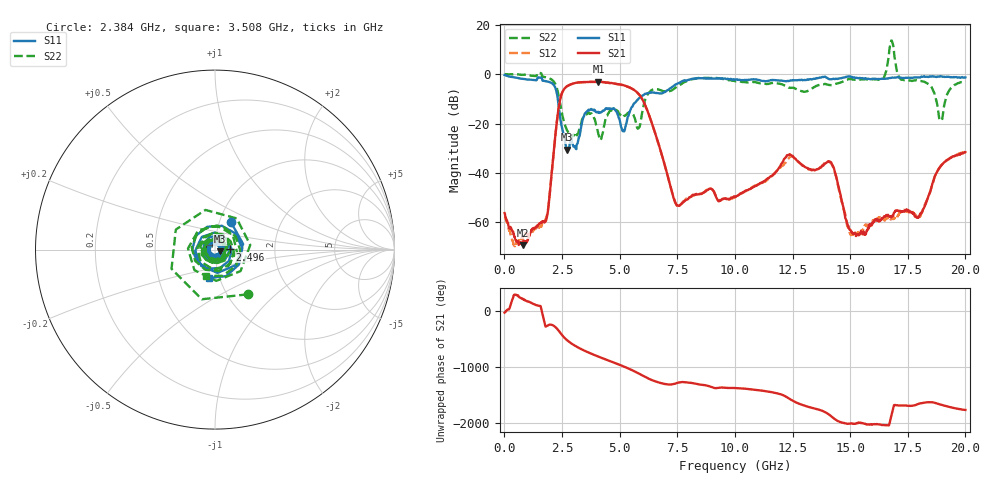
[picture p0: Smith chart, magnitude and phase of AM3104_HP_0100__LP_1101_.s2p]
!Created with skrf (http://scikit-rf.org).
# Hz S RI R 50.0
!freq ReS11 ImS11 ReS21 ImS21 ReS12 ImS12 ReS22 ImS22
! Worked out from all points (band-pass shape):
!   1601 points, 10 MHz to 20 GHz, reference 50 ohm
!   highest |S21| = -3.10 dB at 4.083 GHz (marker M1); lowest = -69.2 dB at 797.1 MHz (marker M2)
!   |S21| within 3 dB of the highest: 2.589 GHz to 5.576 GHz (2.987 GHz wide, 73.2 % of centre)
!   lowest |S11| = -30.6 dB at 2.721 GHz (marker M3), VSWR 1.06, Z = 52.9 - j0.943 ohm
!   |S11| at or under -10 dB: 2.316 GHz to 5.816 GHz (3.5 GHz wide, 86.1 % of centre)
!   |S22| runs from -26.8 to 13.6 dB; largest |S21 - S12| = 0.071
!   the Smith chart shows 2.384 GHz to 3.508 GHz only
!   S11 on the Smith chart (normalised r, x): 2.384 GHz: 1.13, +0.36; 2.496 GHz: 1.18, +0.00; 3.508 GHz: 0.89, -0.29
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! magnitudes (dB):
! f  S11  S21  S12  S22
! 10 MHz  -0.4  -56.3  -57.9  0.0
! 797.1 MHz  -1.9  -69.2  -65.8  -0.2
! 1.822 GHz  -2.9  -58.9  -57.9  -1.3
! 2.384 GHz  -15.0  -12.0  -12.0  -10.2
! 2.496 GHz  -21.6  -7.7  -7.8  -15.8
! 2.721 GHz  -30.6  -4.9  -4.9  -22.8
! 3.346 GHz  -20.5  -3.3  -3.3  -19.5
! 3.508 GHz  -15.8  -3.2  -3.3  -16.2
! 4.083 GHz  -15.3  -3.1  -3.2  -24.5
! 5.17 GHz  -22.8  -4.5  -4.5  -17.1
! 5.782 GHz  -10.4  -7.6  -7.6  -22.0
! 6.682 GHz  -7.8  -28.0  -28.1  -6.2
! 7.506 GHz  -3.9  -53.2  -53.2  -5.0
! 10.01 GHz  -2.3  -49.8  -49.8  -2.9
! 12.33 GHz  -2.8  -32.7  -34.1  -5.5
! 13.34 GHz  -2.1  -38.8  -38.8  -5.8
! 14.2 GHz  -2.1  -36.3  -36.5  -4.4
! 15.05 GHz  -1.1  -63.7  -65.1  -2.0
! 16.68 GHz  -1.6  -57.5  -58.1  7.3
! 18.03 GHz  -1.4  -56.9  -57.7  -2.8
! 18.93 GHz  -0.8  -37.2  -37.2  -18.8
! 20 GHz  -1.3  -31.6  -31.2  -2.8
